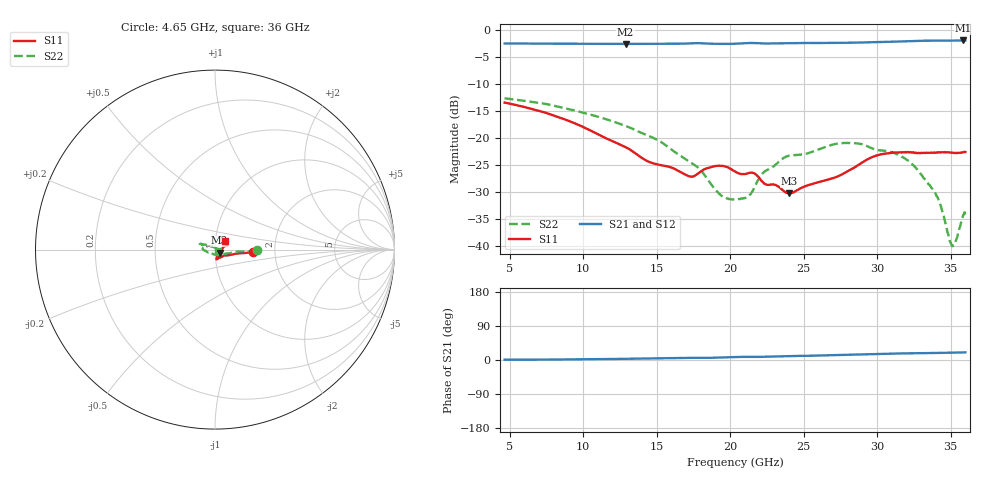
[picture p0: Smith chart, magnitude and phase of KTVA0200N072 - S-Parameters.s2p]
! EMC Technology KTVA0200N072
#HZ S MA R 50
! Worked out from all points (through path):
!   801 points, 4.65 GHz to 36 GHz, reference 50 ohm
!   highest |S21| = -1.94 dB at 35.84 GHz (marker M1); lowest = -2.6 dB at 12.88 GHz (marker M2)
!   lowest |S11| = -30.2 dB at 24.01 GHz (marker M3), VSWR 1.06, Z = 52.6 - j1.8 ohm
!   |S11| at or under -10 dB: start of sweep to end of sweep
!   |S22| runs from -40.0 to -12.7 dB; largest |S21 - S12| = 0.0065
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4.65e9  0.2126 -3.5  0.7484 0.7  0.7502 0.6  0.233 -1.0
9.901125e9  0.1282 -9.5  0.7448 1.8  0.7427 1.9  0.1729 -3.5
1.287938e10  0.0823 -22.6  0.7426 3.1  0.7419 3.1  0.1295 -4.5
1.511306e10  0.05664 -43.0  0.7442 4.1  0.7427 4.2  0.0949 -10.4
1.730756e10  0.04387 -59.7  0.7514 5.7  0.7504 5.8  0.05928 -23.2
1.911019e10  0.05523 -78.3  0.744 6.2  0.7435 6.3  0.03193 -73.2
2.0325e10  0.04894 -79.9  0.7455 7.8  0.7458 7.7  0.02687 -130.5
2.122631e10  0.0472 -71.5  0.7569 8.3  0.7574 8.3  0.02877 -154.0
2.165738e10  0.04695 -74.4  0.7562 8.1  0.7564 8.1  0.03525 -154.4
2.224519e10  0.03867 -70.6  0.7495 8.6  0.7497 8.6  0.0476 -164.8
2.400862e10  0.03077 -33.8  0.7544 10.4  0.7566 10.4  0.06859 -183.3
2.557612e10  0.03754 -11.0  0.7571 11.4  0.7579 11.3  0.07451 -188.6
2.788819e10  0.04844 17.7  0.7612 13.6  0.7612 13.6  0.08989 -198.8
2.957325e10  0.06571 19.2  0.7696 15.3  0.7654 15.1  0.08116 -203.1
3.078806e10  0.07243 22.1  0.7759 16.6  0.7707 16.5  0.07504 -202.1
3.231638e10  0.07347 18.9  0.7894 17.8  0.7849 17.6  0.05831 -207.7
3.384469e10  0.07305 26.5  0.7953 18.4  0.7936 18.5  0.03221 -212.3
3.427575e10  0.07381 30.7  0.7958 18.8  0.7939 18.6  0.02451 -222.1
3.509869e10  0.07304 34.1  0.7969 19.6  0.7946 19.4  0.009975 -287.3
3.533381e10  0.07295 35.8  0.7981 19.8  0.7967 19.7  0.01105 -317.0
3.584325e10  0.0739 39.1  0.7995 20.0  0.8 20.0  0.01922 -362.9
3.6e10  0.07417 38.5  0.7992 20.2  0.7999 20.4  0.01856 -379.5
